| IBIS file created by T2B Version 16.0.0.01291   000
| Cadence Design Systems, Inc. 2011
| This Model is valid for  Temperature Range -40C<=Tc<=125C
| Valid for LPDDR4-1600/2400/3200 operation
| Part Number   VDD2/VDDQ   Package   Architecture
| SCE11N4G320AF   1.1 +0.07/-0.04V   BGA200   16Meg x 16 x 8 x2
| SCE11N8G322AF   1.1 +0.07/-0.04V   BGA200   32Meg x 16 x 8 x2
| SCE11N4G160AF   1.1 +0.07/-0.04V   BGA200   32Meg x 16 x 8 x1
| SCE11N2G160AF   1.1 +0.07/-0.04V   BGA200   16Meg x 16 x 8 x1
| SCE11N2G320AF   1.1 +0.07/-0.04V   BGA200   8Meg x 16 x 8 x2
[IBIS ver] 5.0
[File name]  usesnxxxxaa1.ibs
[File Rev]  1.1
[Date]   2023-09-20
[Source] Simulation of a silicon level SPICE model
[Notes]  IBIS Characteristics for I/O Buffer
   IBIS Model Revision History:
   Rev 1.0:   2020-05-11 - IBIS model file initial creation
   Rev 1.1:   2023-09-20 - update odt data
[Disclaimer]  The IBIS models are for modeling purpose only and are
   subject to change without any notice. UniIC is not
   responsible for any problems the models may cause.
[Copyright] Copyright 2023 UniIC Semiconductors Corp. All rights reserved
|   Component SCE11N4G320AF
[Component] SCE11N4G320AF
[Manufacturer] UniIC Semiconductors Corp.
[Package]
| variable   typ   min   max
R_pkg   1.150   0.687   2.340
L_pkg   1.020nH   0.634nH   2.010nH
C_pkg   0.923pF   0.644pF   3.990pF
[Pin]  signal_name   model_name   R_pin   L_pin   C_pin
A3   VSS   GND   NA   NA   NA
A4   VDD2   POWER   NA   NA   NA
A5   ZQ0   POWER   NA   NA   NA
A9   VDD2   POWER   NA   NA   NA
A10   VSS   GND   NA   NA   NA
A11   ERR_A   ERR   0.862   0.865nH   0.750pF
B2   DQ0_A   DQ   0.711   0.690nH   0.657pF
B3   VDDQ   POWER   NA   NA   NA
B4   DQ7_A   DQ   0.730   0.686nH   0.659pF
B5   VDDQ   POWER   NA   NA   NA
B8   VDDQ   POWER   NA   NA   NA
B9   DQ15_A   DQ   0.702   0.664nH   0.672pF
B10   VDDDQ   POWER   NA   NA   NA
B11   DQ8_A   DQ   0.723   0.706nH   0.669pF
C1   VSS   GND   NA   NA   NA
C2   DQ1_A   DQ   0.687   0.642nH   0.680pF
C3   DMI0_A   DQ   0.822   0.743nH   0.733pF
C4   DQ6_A   DQ   0.704   0.658nH   0.667pF
C5   VSS   GND   NA   NA   NA
C8   VSS   GND   NA   NA   NA
C9   DQ14_A   DQ   0.694   0.654nH   0.669pF
C10   DMI1_A   DQ   0.687   1.080nH   0.781pF
C11   DQ9_A   DQ   1.270   0.643nH   0.670pF
C12   VSS   GND   NA   NA   NA
D1   VDDQ   POWER   NA   NA   NA
D2   VSS   GND   NA   NA   NA
D3   DQS0_T_A   DQ   0.724   0.699nH   0.652pF
D4   VSS   GND   NA   NA   NA
D5   VDDQ   POWER   NA   NA   NA
D8   VDDQ   POWER   NA   NA   NA
D9   VSS   GND   NA   NA   NA
D10   DQS1_T_A   DQ   0.720   0.700nH   0.665pF
D11   VSS   GND   NA   NA   NA
D12   VDDQ   POWER   NA   NA   NA
E1   VSS   GND   NA   NA   NA
E2   DQ2_A   DQ   0.701   0.640nH   0.661pF
E3   DQS0_C_A   DQ   0.735   0.740nH   0.655pF
E4   DQ5_A   DQ   0.732   0.690nH   0.662pF
E5   VSS   GND   NA   NA   NA
E8   VSS   GND   NA   NA   NA
E9   DQ13_A   DQ   0.727   0.687nH   0.670pF
E10   DQS1_C_A   DQ   0.741   0.747nH   0.656pF
E11   DQ10_A   DQ   0.697   0.634nH   0.691pF
E12   VSS   GND   NA   NA   NA
F1   VDD1   POWER   NA   NA   NA
F2   DQ3_A   DQ   0.741   0.703nH   0.646pF
F3   VDDQ   POWER   NA   NA   NA
F4   DQ4_A   DQ   0.729   0.671nH   0.649pF
F5   VDD2   POWER   NA   NA   NA
F8   VDD2   POWER   NA   NA   NA
F9   DQ12_A   DQ   1.100   0.858nH   0.709pF
F10   VDDQ   POWER   NA   NA   NA
F11   DQ11_A   DQ   0.728   0.685nH   0.658pF
F12   VDD1   POWER   NA   NA   NA
G1   VSS   GND   NA   NA   NA
G2   ODT_CA_A   PINEN   1.660   1.430nH   1.024pF
G3   VSS   GND   NA   NA   NA
G4   VDD1   POWER   NA   NA   NA
G5   VSS   GND   NA   NA   NA
G8   VSS   GND   NA   NA   NA
G9   VDD1   POWER   NA   NA   NA
G10   VSS   GND   NA   NA   NA
G12   VSS   GND   NA   NA   NA
H1   VDD2   POWER   NA   NA   NA
H2   CA0_A   CLKCA   2.000   1.690nH   1.170pF
H4   CS0_A   CLKCA   1.680   1.430nH   1.070pF
H5   VDD2   POWER   NA   NA   NA
H8   VDD2   POWER   NA   NA   NA
H9   CA2_A   CLKCA   1.960   1.660nH   1.160pF
H10   CA3_A   CLKCA   1.940   1.640nH   1.170pF
H11   CA4_A   CLKCA   2.020   1.700nH   1.200pF
H12   VDD2   POWER   NA   NA   NA
J1   VSS   GND   NA   NA   NA
J2   CA1_A   CLKCA   2.000   1.680nH   1.160pF
J3   VSS   GND   NA   NA   NA
J4   CKE0_A   PINEN   1.600   1.380nH   1.000pF
J8   CK_T_A   CLKCA   1.720   1.510nH   1.050pF
J9   CK_C_A   CLKCA   1.740   1.543nH   1.050pF
J10   VSS   GND   NA   NA   NA
J11   CA5_A   CLKCA   2.030   1.690nH   1.200pF
J12   VSS   GND   NA   NA   NA
K1   VDD2   POWER   NA   NA   NA
K2   VSS   GND   NA   NA   NA
K3   VDD2   POWER   NA   NA   NA
K4   VSS   GND   NA   NA   NA
K9   VSS   GND   NA   NA   NA
K10   VDD2   POWER   NA   NA   NA
K11   VSS   GND   NA   NA   NA
K12   VDD2   POWER   NA   NA   NA
N1   VDD2   POWER   NA   NA   NA
N2   VSS   GND   NA   NA   NA
N3   VDD2   POWER   NA   NA   NA
N4   VSS   GND   NA   NA   NA
N9   VSS   GND   NA   NA   NA
N10   VDD2   POWER   NA   NA   NA
N11   VSS   GND   NA   NA   NA
N12   VDD2   POWER   NA   NA   NA
P1   VSS   GND   NA   NA   NA
P2   CA1_B   CLKCA   2.000   1.690nH   1.160pF
P3   VSS   GND   NA   NA   NA
P4   CKE0_B   PINEN   1.600   1.390nH   0.999pF
P8   CK_T_B   CLKCA   1.740   1.510nH   1.060pF
P9   CK_C_B   CLKCA   1.740   1.530nH   1.050pF
P10   VSS   GND   NA   NA   NA
P11   CA5_B   CLKCA   2.030   1.710nH   1.180pF
P12   VSS   GND   NA   NA   NA
R1   VDD2   POWER   NA   NA   NA
R2   CA0_B   CLKCA   2.000   1.690nH   1.170pF
R4   CS0_B   CLKCA   1.680   1.430nH   1.070pF
R5   VDD2   POWER   NA   NA   NA
R8   VDD2   POWER   NA   NA   NA
R9   CA2_B   CLKCA   2.000   1.700nH   1.180pF
R10   CA3_B   CLKCA   1.930   1.630nH   1.170pF
R11   CA4_B   CLKCA   1.980   1.680nH   1.190pF
R12   VDD2   POWER   NA   NA   NA
T1   VSS   GND   NA   NA   NA
T2   ODT_CA_B   PINEN   2.020   1.598nH   1.079pF
T3   VSS   GND   NA   NA   NA
T4   VDD1   POWER   NA   NA   NA
T5   VSS   GND   NA   NA   NA
T8   VSS   GND   NA   NA   NA
T9   VDD1   POWER   NA   NA   NA
T10   VSS   GND   NA   NA   NA
T11   RESET_N   PINEN   2.020   1.598nH   1.079pF
T12   VSS   GND   NA   NA   NA
U1   VDD1   POWER   NA   NA   NA
U2   DQ3_B   DQ   1.110   0.889nH   0.704pF
U3   VDDQ   POWER   NA   NA   NA
U4   DQ4_B   DQ   1.080   0.845nH   0.704pF
U5   VDD2   POWER   NA   NA   NA
U8   VDD2   POWER   NA   NA   NA
U9   DQ12_B   DQ   0.727   0.672nH   0.654pF
U10   VDDQ   POWER   NA   NA   NA
U11   DQ11_B   DQ   0.749   0.707nH   0.644pF
U12   VDD1   POWER   NA   NA   NA
V1   VSS   GND   NA   NA   NA
V2   DQ2_B   DQ   0.704   0.646nH   0.659pF
V3   DQS0_C_B   DQ   0.738   0.745nH   0.673pF
V4   DQ5_B   DQ   0.723   0.684nH   0.677pF
V5   VSS   GND   NA   NA   NA
V8   VSS   GND   NA   NA   NA
V9   DQ13_B   DQ   0.722   0.685nH   0.673pF
V10   DQS1_C_B   DQ   0.738   0.747nH   0.647pF
V11   DQ10_B   DQ   0.696   0.645nH   0.666pF
V12   VSS   GND   NA   NA   NA
W1   VDDQ   POWER   NA   NA   NA
W2   VSS   GND   NA   NA   NA
W3   DQS0_T_B   DQ   0.734   0.716nH   0.652pF
W4   VSS   GND   NA   NA   NA
W5   VDDQ   POWER   NA   NA   NA
W8   VDDQ   POWER   NA   NA   NA
W9   VSS   GND   NA   NA   NA
W10   DQS1_T_B   DQ   0.731   0.708nH   0.656pF
W11   VSS   GND   NA   NA   NA
W12   VDDQ   POWER   NA   NA   NA
Y1   VSS   GND   NA   NA   NA
Y2   DQ1_B   DQ   1.130   0.969nH   0.723pF
Y3   DMI0_B   DQ   0.820   0.739nH   0.734pF
Y4   DQ6_B   DQ   0.698   0.655nH   0.668pF
Y5   VSS   GND   NA   NA   NA
Y8   VSS   GND   NA   NA   NA
Y9   DQ14_B   DQ   0.691   0.653nH   0.672pF
Y10   DMI1_B   DQ   0.819   0.738nH   0.735pF
Y11   DQ9_B   DQ   0.688   0.642nH   0.676pF
Y12   VSS   GND   NA   NA   NA
AA2   DQ0_B   DQ   0.709   0.697nH   0.668pF
AA3   VDDQ   POWER   NA   NA   NA
AA4   DQ7_B   DQ   0.735   0.700nH   0.660pF
AA5   VDDQ   POWER   NA   NA   NA
AA8   VDDQ   POWER   NA   NA   NA
AA9   DQ15_B   DQ   0.709   0.666nH   0.683pF
AA10   VDDQ   POWER   NA   NA   NA
AA11   DQ8_B   DQ   0.716   0.695nH   0.675pF
AB3   VSS   GND   NA   NA   NA
AB4   VDD2   POWER   NA   NA   NA
AB5   VSS   GND   NA   NA   NA
AB8   VSS   GND   NA   NA   NA
AB9   VDD2   POWER   NA   NA   NA
AB10   VSS   GND   NA   NA   NA
AB11   ERR_B   ERR   2.340   2.010nH   3.990pF
|IN   dq_in   dummy
|EN   dq_en   dummy
[Diff pin]  inv_pin  vdiff   tdelay_typ   tdelay_min   tdelay_max
D3   E3   0.180V   NA   NA   NA
D10   E10   0.180V   NA   NA   NA
J8   J9   0.180V   NA   NA   NA
P8   P9   0.180V   NA   NA   NA
W3   V3   0.180V   NA   NA   NA
W10   V10   0.180V   NA   NA   NA
|   Component SCE11N8G322AF
[Component] SCE11N8G322AF
[Manufacturer] UniIC Semiconductors Corp.
[Package]
| variable   typ   min   max
R_pkg   1.150   0.687   2.340
L_pkg   1.020nH   0.634nH   2.010nH
C_pkg   0.923pF   0.644pF   3.990pF
[Pin]  signal_name   model_name   R_pin   L_pin   C_pin
A3   VSS   GND   NA   NA   NA
A4   VDD2   POWER   NA   NA   NA
A5   ZQ0   POWER   NA   NA   NA
A9   VDD2   POWER   NA   NA   NA
A10   VSS   GND   NA   NA   NA
A11   ERR_A   ERR   0.862   0.865nH   0.750pF
B2   DQ0_A   DQ   0.711   0.690nH   0.657pF
B3   VDDQ   POWER   NA   NA   NA
B4   DQ7_A   DQ   0.730   0.686nH   0.659pF
B5   VDDQ   POWER   NA   NA   NA
B8   VDDQ   POWER   NA   NA   NA
B9   DQ15_A   DQ   0.702   0.664nH   0.672pF
B10   VDDDQ   POWER   NA   NA   NA
B11   DQ8_A   DQ   0.723   0.706nH   0.669pF
C1   VSS   GND   NA   NA   NA
C2   DQ1_A   DQ   0.687   0.642nH   0.680pF
C3   DMI0_A   DQ   0.822   0.743nH   0.733pF
C4   DQ6_A   DQ   0.704   0.658nH   0.667pF
C5   VSS   GND   NA   NA   NA
C8   VSS   GND   NA   NA   NA
C9   DQ14_A   DQ   0.694   0.654nH   0.669pF
C10   DMI1_A   DQ   0.687   1.080nH   0.781pF
C11   DQ9_A   DQ   1.270   0.643nH   0.670pF
C12   VSS   GND   NA   NA   NA
D1   VDDQ   POWER   NA   NA   NA
D2   VSS   GND   NA   NA   NA
D3   DQS0_T_A   DQ   0.724   0.699nH   0.652pF
D4   VSS   GND   NA   NA   NA
D5   VDDQ   POWER   NA   NA   NA
D8   VDDQ   POWER   NA   NA   NA
D9   VSS   GND   NA   NA   NA
D10   DQS1_T_A   DQ   0.720   0.700nH   0.665pF
D11   VSS   GND   NA   NA   NA
D12   VDDQ   POWER   NA   NA   NA
E1   VSS   GND   NA   NA   NA
E2   DQ2_A   DQ   0.701   0.640nH   0.661pF
E3   DQS0_C_A   DQ   0.735   0.740nH   0.655pF
E4   DQ5_A   DQ   0.732   0.690nH   0.662pF
E5   VSS   GND   NA   NA   NA
E8   VSS   GND   NA   NA   NA
E9   DQ13_A   DQ   0.727   0.687nH   0.670pF
E10   DQS1_C_A   DQ   0.741   0.747nH   0.656pF
E11   DQ10_A   DQ   0.697   0.634nH   0.691pF
E12   VSS   GND   NA   NA   NA
F1   VDD1   POWER   NA   NA   NA
F2   DQ3_A   DQ   0.741   0.703nH   0.646pF
F3   VDDQ   POWER   NA   NA   NA
F4   DQ4_A   DQ   0.729   0.671nH   0.649pF
F5   VDD2   POWER   NA   NA   NA
F8   VDD2   POWER   NA   NA   NA
F9   DQ12_A   DQ   1.100   0.858nH   0.709pF
F10   VDDQ   POWER   NA   NA   NA
F11   DQ11_A   DQ   0.728   0.685nH   0.658pF
F12   VDD1   POWER   NA   NA   NA
G1   VSS   GND   NA   NA   NA
G2   ODT_CA_A   PINEN   1.660   1.430nH   1.024pF
G3   VSS   GND   NA   NA   NA
G4   VDD1   POWER   NA   NA   NA
G5   VSS   GND   NA   NA   NA
G8   VSS   GND   NA   NA   NA
G9   VDD1   POWER   NA   NA   NA
G10   VSS   GND   NA   NA   NA
G12   VSS   GND   NA   NA   NA
H1   VDD2   POWER   NA   NA   NA
H2   CA0_A   CLKCA   2.000   1.690nH   1.170pF
H4   CS0_A   CLKCA   1.680   1.430nH   1.070pF
H5   VDD2   POWER   NA   NA   NA
H8   VDD2   POWER   NA   NA   NA
H9   CA2_A   CLKCA   1.960   1.660nH   1.160pF
H10   CA3_A   CLKCA   1.940   1.640nH   1.170pF
H11   CA4_A   CLKCA   2.020   1.700nH   1.200pF
H12   VDD2   POWER   NA   NA   NA
J1   VSS   GND   NA   NA   NA
J2   CA1_A   CLKCA   2.000   1.680nH   1.160pF
J3   VSS   GND   NA   NA   NA
J4   CKE0_A   PINEN   1.600   1.380nH   1.000pF
J8   CK_T_A   CLKCA   1.720   1.510nH   1.050pF
J9   CK_C_A   CLKCA   1.740   1.543nH   1.050pF
J10   VSS   GND   NA   NA   NA
J11   CA5_A   CLKCA   2.030   1.690nH   1.200pF
J12   VSS   GND   NA   NA   NA
K1   VDD2   POWER   NA   NA   NA
K2   VSS   GND   NA   NA   NA
K3   VDD2   POWER   NA   NA   NA
K4   VSS   GND   NA   NA   NA
K9   VSS   GND   NA   NA   NA
K10   VDD2   POWER   NA   NA   NA
K11   VSS   GND   NA   NA   NA
K12   VDD2   POWER   NA   NA   NA
N1   VDD2   POWER   NA   NA   NA
N2   VSS   GND   NA   NA   NA
N3   VDD2   POWER   NA   NA   NA
N4   VSS   GND   NA   NA   NA
N9   VSS   GND   NA   NA   NA
N10   VDD2   POWER   NA   NA   NA
N11   VSS   GND   NA   NA   NA
N12   VDD2   POWER   NA   NA   NA
P1   VSS   GND   NA   NA   NA
P2   CA1_B   CLKCA   2.000   1.690nH   1.160pF
P3   VSS   GND   NA   NA   NA
P4   CKE0_B   PINEN   1.600   1.390nH   0.999pF
P8   CK_T_B   CLKCA   1.740   1.510nH   1.060pF
P9   CK_C_B   CLKCA   1.740   1.530nH   1.050pF
P10   VSS   GND   NA   NA   NA
P11   CA5_B   CLKCA   2.030   1.710nH   1.180pF
P12   VSS   GND   NA   NA   NA
R1   VDD2   POWER   NA   NA   NA
R2   CA0_B   CLKCA   2.000   1.690nH   1.170pF
R4   CS0_B   CLKCA   1.680   1.430nH   1.070pF
R5   VDD2   POWER   NA   NA   NA
R8   VDD2   POWER   NA   NA   NA
R9   CA2_B   CLKCA   2.000   1.700nH   1.180pF
R10   CA3_B   CLKCA   1.930   1.630nH   1.170pF
R11   CA4_B   CLKCA   1.980   1.680nH   1.190pF
R12   VDD2   POWER   NA   NA   NA
T1   VSS   GND   NA   NA   NA
T2   ODT_CA_B   PINEN   2.020   1.598nH   1.079pF
T3   VSS   GND   NA   NA   NA
T4   VDD1   POWER   NA   NA   NA
T5   VSS   GND   NA   NA   NA
T8   VSS   GND   NA   NA   NA
T9   VDD1   POWER   NA   NA   NA
T10   VSS   GND   NA   NA   NA
T11   RESET_N   PINEN   2.020   1.598nH   1.079pF
T12   VSS   GND   NA   NA   NA
U1   VDD1   POWER   NA   NA   NA
U2   DQ3_B   DQ   1.110   0.889nH   0.704pF
U3   VDDQ   POWER   NA   NA   NA
U4   DQ4_B   DQ   1.080   0.845nH   0.704pF
U5   VDD2   POWER   NA   NA   NA
U8   VDD2   POWER   NA   NA   NA
U9   DQ12_B   DQ   0.727   0.672nH   0.654pF
U10   VDDQ   POWER   NA   NA   NA
U11   DQ11_B   DQ   0.749   0.707nH   0.644pF
U12   VDD1   POWER   NA   NA   NA
V1   VSS   GND   NA   NA   NA
V2   DQ2_B   DQ   0.704   0.646nH   0.659pF
V3   DQS0_C_B   DQ   0.738   0.745nH   0.673pF
V4   DQ5_B   DQ   0.723   0.684nH   0.677pF
V5   VSS   GND   NA   NA   NA
V8   VSS   GND   NA   NA   NA
V9   DQ13_B   DQ   0.722   0.685nH   0.673pF
V10   DQS1_C_B   DQ   0.738   0.747nH   0.647pF
V11   DQ10_B   DQ   0.696   0.645nH   0.666pF
V12   VSS   GND   NA   NA   NA
W1   VDDQ   POWER   NA   NA   NA
W2   VSS   GND   NA   NA   NA
W3   DQS0_T_B   DQ   0.734   0.716nH   0.652pF
W4   VSS   GND   NA   NA   NA
W5   VDDQ   POWER   NA   NA   NA
W8   VDDQ   POWER   NA   NA   NA
W9   VSS   GND   NA   NA   NA
W10   DQS1_T_B   DQ   0.731   0.708nH   0.656pF
W11   VSS   GND   NA   NA   NA
W12   VDDQ   POWER   NA   NA   NA
Y1   VSS   GND   NA   NA   NA
Y2   DQ1_B   DQ   1.130   0.969nH   0.723pF
Y3   DMI0_B   DQ   0.820   0.739nH   0.734pF
Y4   DQ6_B   DQ   0.698   0.655nH   0.668pF
Y5   VSS   GND   NA   NA   NA
Y8   VSS   GND   NA   NA   NA
Y9   DQ14_B   DQ   0.691   0.653nH   0.672pF
Y10   DMI1_B   DQ   0.819   0.738nH   0.735pF
Y11   DQ9_B   DQ   0.688   0.642nH   0.676pF
Y12   VSS   GND   NA   NA   NA
AA2   DQ0_B   DQ   0.709   0.697nH   0.668pF
AA3   VDDQ   POWER   NA   NA   NA
AA4   DQ7_B   DQ   0.735   0.700nH   0.660pF
AA5   VDDQ   POWER   NA   NA   NA
AA8   VDDQ   POWER   NA   NA   NA
AA9   DQ15_B   DQ   0.709   0.666nH   0.683pF
AA10   VDDQ   POWER   NA   NA   NA
AA11   DQ8_B   DQ   0.716   0.695nH   0.675pF
AB3   VSS   GND   NA   NA   NA
AB4   VDD2   POWER   NA   NA   NA
AB5   VSS   GND   NA   NA   NA
AB8   VSS   GND   NA   NA   NA
AB9   VDD2   POWER   NA   NA   NA
AB10   VSS   GND   NA   NA   NA
AB11   ERR_B   ERR   2.340   2.010nH   3.990pF
|IN   dq_in   dummy
|EN   dq_en   dummy
[Diff pin]  inv_pin  vdiff   tdelay_typ   tdelay_min   tdelay_max
D3   E3   0.180V   NA   NA   NA
D10   E10   0.180V   NA   NA   NA
J8   J9   0.180V   NA   NA   NA
P8   P9   0.180V   NA   NA   NA
W3   V3   0.180V   NA   NA   NA
W10   V10   0.180V   NA   NA   NA
|   Component SCE11N4G160AF
[Component] SCE11N4G160AF
[Manufacturer] UniIC Semiconductors Corp.
[Package]
| variable   typ   min   max
R_pkg   1.150   0.687   2.340
L_pkg   1.020nH   0.634nH   2.010nH
C_pkg   0.923pF   0.644pF   3.990pF
[Pin]  signal_name   model_name   R_pin   L_pin   C_pin
A3   VSS   GND   NA   NA   NA
A4   VDD2   POWER   NA   NA   NA
A5   ZQ0   POWER   NA   NA   NA
A9   VDD2   POWER   NA   NA   NA
A10   VSS   GND   NA   NA   NA
A11   ERR_A   ERR   0.862   0.865nH   0.750pF
B2   DQ0_A   DQ   0.711   0.690nH   0.657pF
B3   VDDQ   POWER   NA   NA   NA
B4   DQ7_A   DQ   0.730   0.686nH   0.659pF
B5   VDDQ   POWER   NA   NA   NA
B8   VDDQ   POWER   NA   NA   NA
B9   DQ15_A   DQ   0.702   0.664nH   0.672pF
B10   VDDDQ   POWER   NA   NA   NA
B11   DQ8_A   DQ   0.723   0.706nH   0.669pF
C1   VSS   GND   NA   NA   NA
C2   DQ1_A   DQ   0.687   0.642nH   0.680pF
C3   DMI0_A   DQ   0.822   0.743nH   0.733pF
C4   DQ6_A   DQ   0.704   0.658nH   0.667pF
C5   VSS   GND   NA   NA   NA
C8   VSS   GND   NA   NA   NA
C9   DQ14_A   DQ   0.694   0.654nH   0.669pF
C10   DMI1_A   DQ   0.687   1.080nH   0.781pF
C11   DQ9_A   DQ   1.270   0.643nH   0.670pF
C12   VSS   GND   NA   NA   NA
D1   VDDQ   POWER   NA   NA   NA
D2   VSS   GND   NA   NA   NA
D3   DQS0_T_A   DQ   0.724   0.699nH   0.652pF
D4   VSS   GND   NA   NA   NA
D5   VDDQ   POWER   NA   NA   NA
D8   VDDQ   POWER   NA   NA   NA
D9   VSS   GND   NA   NA   NA
D10   DQS1_T_A   DQ   0.720   0.700nH   0.665pF
D11   VSS   GND   NA   NA   NA
D12   VDDQ   POWER   NA   NA   NA
E1   VSS   GND   NA   NA   NA
E2   DQ2_A   DQ   0.701   0.640nH   0.661pF
E3   DQS0_C_A   DQ   0.735   0.740nH   0.655pF
E4   DQ5_A   DQ   0.732   0.690nH   0.662pF
E5   VSS   GND   NA   NA   NA
E8   VSS   GND   NA   NA   NA
E9   DQ13_A   DQ   0.727   0.687nH   0.670pF
E10   DQS1_C_A   DQ   0.741   0.747nH   0.656pF
E11   DQ10_A   DQ   0.697   0.634nH   0.691pF
E12   VSS   GND   NA   NA   NA
F1   VDD1   POWER   NA   NA   NA
F2   DQ3_A   DQ   0.741   0.703nH   0.646pF
F3   VDDQ   POWER   NA   NA   NA
F4   DQ4_A   DQ   0.729   0.671nH   0.649pF
F5   VDD2   POWER   NA   NA   NA
F8   VDD2   POWER   NA   NA   NA
F9   DQ12_A   DQ   1.100   0.858nH   0.709pF
F10   VDDQ   POWER   NA   NA   NA
F11   DQ11_A   DQ   0.728   0.685nH   0.658pF
F12   VDD1   POWER   NA   NA   NA
G1   VSS   GND   NA   NA   NA
G2   ODT_CA_A   PINEN   1.660   1.430nH   1.024pF
G3   VSS   GND   NA   NA   NA
G4   VDD1   POWER   NA   NA   NA
G5   VSS   GND   NA   NA   NA
G8   VSS   GND   NA   NA   NA
G9   VDD1   POWER   NA   NA   NA
G10   VSS   GND   NA   NA   NA
G12   VSS   GND   NA   NA   NA
H1   VDD2   POWER   NA   NA   NA
H2   CA0_A   CLKCA   2.000   1.690nH   1.170pF
H4   CS0_A   CLKCA   1.680   1.430nH   1.070pF
H5   VDD2   POWER   NA   NA   NA
H8   VDD2   POWER   NA   NA   NA
H9   CA2_A   CLKCA   1.960   1.660nH   1.160pF
H10   CA3_A   CLKCA   1.940   1.640nH   1.170pF
H11   CA4_A   CLKCA   2.020   1.700nH   1.200pF
H12   VDD2   POWER   NA   NA   NA
J1   VSS   GND   NA   NA   NA
J2   CA1_A   CLKCA   2.000   1.680nH   1.160pF
J3   VSS   GND   NA   NA   NA
J4   CKE0_A   PINEN   1.600   1.380nH   1.000pF
J8   CK_T_A   CLKCA   1.720   1.510nH   1.050pF
J9   CK_C_A   CLKCA   1.740   1.543nH   1.050pF
J10   VSS   GND   NA   NA   NA
J11   CA5_A   CLKCA   2.030   1.690nH   1.200pF
J12   VSS   GND   NA   NA   NA
K1   VDD2   POWER   NA   NA   NA
K2   VSS   GND   NA   NA   NA
K3   VDD2   POWER   NA   NA   NA
K4   VSS   GND   NA   NA   NA
K9   VSS   GND   NA   NA   NA
K10   VDD2   POWER   NA   NA   NA
K11   VSS   GND   NA   NA   NA
K12   VDD2   POWER   NA   NA   NA
N1   VDD2   POWER   NA   NA   NA
N2   VSS   GND   NA   NA   NA
N3   VDD2   POWER   NA   NA   NA
N4   VSS   GND   NA   NA   NA
N9   VSS   GND   NA   NA   NA
N10   VDD2   POWER   NA   NA   NA
N11   VSS   GND   NA   NA   NA
N12   VDD2   POWER   NA   NA   NA
P1   VSS   GND   NA   NA   NA
P3   VSS   GND   NA   NA   NA
P10   VSS   GND   NA   NA   NA
P12   VSS   GND   NA   NA   NA
R1   VDD2   POWER   NA   NA   NA
R5   VDD2   POWER   NA   NA   NA
R8   VDD2   POWER   NA   NA   NA
R12   VDD2   POWER   NA   NA   NA
T1   VSS   GND   NA   NA   NA
T3   VSS   GND   NA   NA   NA
T4   VDD1   POWER   NA   NA   NA
T5   VSS   GND   NA   NA   NA
T8   VSS   GND   NA   NA   NA
T9   VDD1   POWER   NA   NA   NA
T10   VSS   GND   NA   NA   NA
T11   RESET_N   PINEN   2.020   1.598nH   1.079pF
T12   VSS   GND   NA   NA   NA
U1   VDD1   POWER   NA   NA   NA
U3   VDDQ   POWER   NA   NA   NA
U5   VDD2   POWER   NA   NA   NA
U8   VDD2   POWER   NA   NA   NA
U10   VDDQ   POWER   NA   NA   NA
U12   VDD1   POWER   NA   NA   NA
V1   VSS   GND   NA   NA   NA
V5   VSS   GND   NA   NA   NA
V8   VSS   GND   NA   NA   NA
V12   VSS   GND   NA   NA   NA
W1   VDDQ   POWER   NA   NA   NA
W2   VSS   GND   NA   NA   NA
W4   VSS   GND   NA   NA   NA
W5   VDDQ   POWER   NA   NA   NA
W8   VDDQ   POWER   NA   NA   NA
W9   VSS   GND   NA   NA   NA
W11   VSS   GND   NA   NA   NA
W12   VDDQ   POWER   NA   NA   NA
Y1   VSS   GND   NA   NA   NA
Y5   VSS   GND   NA   NA   NA
Y8   VSS   GND   NA   NA   NA
Y12   VSS   GND   NA   NA   NA
AA3   VDDQ   POWER   NA   NA   NA
AA5   VDDQ   POWER   NA   NA   NA
AA8   VDDQ   POWER   NA   NA   NA
AA10   VDDQ   POWER   NA   NA   NA
AB3   VSS   GND   NA   NA   NA
AB4   VDD2   POWER   NA   NA   NA
AB5   VSS   GND   NA   NA   NA
AB8   VSS   GND   NA   NA   NA
AB9   VDD2   POWER   NA   NA   NA
AB10   VSS   GND   NA   NA   NA
|IN   dq_in   dummy
|EN   dq_en   dummy
[Diff pin]  inv_pin  vdiff   tdelay_typ   tdelay_min   tdelay_max
D3   E3   0.180V   NA   NA   NA
D10   E10   0.180V   NA   NA   NA
J8   J9   0.180V   NA   NA   NA
|   Component SCE11N2G160AF
[Component] SCE11N2G160AF
[Manufacturer] UniIC Semiconductors Corp.
[Package]
| variable   typ   min   max
R_pkg   1.150   0.687   2.340
L_pkg   1.020nH   0.634nH   2.010nH
C_pkg   0.923pF   0.644pF   3.990pF
[Pin]  signal_name   model_name   R_pin   L_pin   C_pin
A3   VSS   GND   NA   NA   NA
A4   VDD2   POWER   NA   NA   NA
A5   ZQ0   POWER   NA   NA   NA
A9   VDD2   POWER   NA   NA   NA
A10   VSS   GND   NA   NA   NA
A11   ERR_A   ERR   0.862   0.865nH   0.750pF
B2   DQ0_A   DQ   0.711   0.690nH   0.657pF
B3   VDDQ   POWER   NA   NA   NA
B4   DQ7_A   DQ   0.730   0.686nH   0.659pF
B5   VDDQ   POWER   NA   NA   NA
B8   VDDQ   POWER   NA   NA   NA
B9   DQ15_A   DQ   0.702   0.664nH   0.672pF
B10   VDDDQ   POWER   NA   NA   NA
B11   DQ8_A   DQ   0.723   0.706nH   0.669pF
C1   VSS   GND   NA   NA   NA
C2   DQ1_A   DQ   0.687   0.642nH   0.680pF
C3   DMI0_A   DQ   0.822   0.743nH   0.733pF
C4   DQ6_A   DQ   0.704   0.658nH   0.667pF
C5   VSS   GND   NA   NA   NA
C8   VSS   GND   NA   NA   NA
C9   DQ14_A   DQ   0.694   0.654nH   0.669pF
C10   DMI1_A   DQ   0.687   1.080nH   0.781pF
C11   DQ9_A   DQ   1.270   0.643nH   0.670pF
C12   VSS   GND   NA   NA   NA
D1   VDDQ   POWER   NA   NA   NA
D2   VSS   GND   NA   NA   NA
D3   DQS0_T_A   DQ   0.724   0.699nH   0.652pF
D4   VSS   GND   NA   NA   NA
D5   VDDQ   POWER   NA   NA   NA
D8   VDDQ   POWER   NA   NA   NA
D9   VSS   GND   NA   NA   NA
D10   DQS1_T_A   DQ   0.720   0.700nH   0.665pF
D11   VSS   GND   NA   NA   NA
D12   VDDQ   POWER   NA   NA   NA
E1   VSS   GND   NA   NA   NA
E2   DQ2_A   DQ   0.701   0.640nH   0.661pF
E3   DQS0_C_A   DQ   0.735   0.740nH   0.655pF
E4   DQ5_A   DQ   0.732   0.690nH   0.662pF
E5   VSS   GND   NA   NA   NA
E8   VSS   GND   NA   NA   NA
E9   DQ13_A   DQ   0.727   0.687nH   0.670pF
E10   DQS1_C_A   DQ   0.741   0.747nH   0.656pF
E11   DQ10_A   DQ   0.697   0.634nH   0.691pF
E12   VSS   GND   NA   NA   NA
F1   VDD1   POWER   NA   NA   NA
F2   DQ3_A   DQ   0.741   0.703nH   0.646pF
F3   VDDQ   POWER   NA   NA   NA
F4   DQ4_A   DQ   0.729   0.671nH   0.649pF
F5   VDD2   POWER   NA   NA   NA
F8   VDD2   POWER   NA   NA   NA
F9   DQ12_A   DQ   1.100   0.858nH   0.709pF
F10   VDDQ   POWER   NA   NA   NA
F11   DQ11_A   DQ   0.728   0.685nH   0.658pF
F12   VDD1   POWER   NA   NA   NA
G1   VSS   GND   NA   NA   NA
G2   ODT_CA_A   PINEN   1.660   1.430nH   1.024pF
G3   VSS   GND   NA   NA   NA
G4   VDD1   POWER   NA   NA   NA
G5   VSS   GND   NA   NA   NA
G8   VSS   GND   NA   NA   NA
G9   VDD1   POWER   NA   NA   NA
G10   VSS   GND   NA   NA   NA
G12   VSS   GND   NA   NA   NA
H1   VDD2   POWER   NA   NA   NA
H2   CA0_A   CLKCA   2.000   1.690nH   1.170pF
H4   CS0_A   CLKCA   1.680   1.430nH   1.070pF
H5   VDD2   POWER   NA   NA   NA
H8   VDD2   POWER   NA   NA   NA
H9   CA2_A   CLKCA   1.960   1.660nH   1.160pF
H10   CA3_A   CLKCA   1.940   1.640nH   1.170pF
H11   CA4_A   CLKCA   2.020   1.700nH   1.200pF
H12   VDD2   POWER   NA   NA   NA
J1   VSS   GND   NA   NA   NA
J2   CA1_A   CLKCA   2.000   1.680nH   1.160pF
J3   VSS   GND   NA   NA   NA
J4   CKE0_A   PINEN   1.600   1.380nH   1.000pF
J8   CK_T_A   CLKCA   1.720   1.510nH   1.050pF
J9   CK_C_A   CLKCA   1.740   1.543nH   1.050pF
J10   VSS   GND   NA   NA   NA
J11   CA5_A   CLKCA   2.030   1.690nH   1.200pF
J12   VSS   GND   NA   NA   NA
K1   VDD2   POWER   NA   NA   NA
K2   VSS   GND   NA   NA   NA
K3   VDD2   POWER   NA   NA   NA
K4   VSS   GND   NA   NA   NA
K9   VSS   GND   NA   NA   NA
K10   VDD2   POWER   NA   NA   NA
K11   VSS   GND   NA   NA   NA
K12   VDD2   POWER   NA   NA   NA
N1   VDD2   POWER   NA   NA   NA
N2   VSS   GND   NA   NA   NA
N3   VDD2   POWER   NA   NA   NA
N4   VSS   GND   NA   NA   NA
N9   VSS   GND   NA   NA   NA
N10   VDD2   POWER   NA   NA   NA
N11   VSS   GND   NA   NA   NA
N12   VDD2   POWER   NA   NA   NA
P1   VSS   GND   NA   NA   NA
P3   VSS   GND   NA   NA   NA
P10   VSS   GND   NA   NA   NA
P12   VSS   GND   NA   NA   NA
R1   VDD2   POWER   NA   NA   NA
R5   VDD2   POWER   NA   NA   NA
R8   VDD2   POWER   NA   NA   NA
R12   VDD2   POWER   NA   NA   NA
T1   VSS   GND   NA   NA   NA
T3   VSS   GND   NA   NA   NA
T4   VDD1   POWER   NA   NA   NA
T5   VSS   GND   NA   NA   NA
T8   VSS   GND   NA   NA   NA
T9   VDD1   POWER   NA   NA   NA
T10   VSS   GND   NA   NA   NA
T11   RESET_N   PINEN   2.020   1.598nH   1.079pF
T12   VSS   GND   NA   NA   NA
U1   VDD1   POWER   NA   NA   NA
U3   VDDQ   POWER   NA   NA   NA
U5   VDD2   POWER   NA   NA   NA
U8   VDD2   POWER   NA   NA   NA
U10   VDDQ   POWER   NA   NA   NA
U12   VDD1   POWER   NA   NA   NA
V1   VSS   GND   NA   NA   NA
V5   VSS   GND   NA   NA   NA
V8   VSS   GND   NA   NA   NA
V12   VSS   GND   NA   NA   NA
W1   VDDQ   POWER   NA   NA   NA
W2   VSS   GND   NA   NA   NA
W4   VSS   GND   NA   NA   NA
W5   VDDQ   POWER   NA   NA   NA
W8   VDDQ   POWER   NA   NA   NA
W9   VSS   GND   NA   NA   NA
W11   VSS   GND   NA   NA   NA
W12   VDDQ   POWER   NA   NA   NA
Y1   VSS   GND   NA   NA   NA
Y5   VSS   GND   NA   NA   NA
Y8   VSS   GND   NA   NA   NA
Y12   VSS   GND   NA   NA   NA
AA3   VDDQ   POWER   NA   NA   NA
AA5   VDDQ   POWER   NA   NA   NA
AA8   VDDQ   POWER   NA   NA   NA
AA10   VDDQ   POWER   NA   NA   NA
AB3   VSS   GND   NA   NA   NA
AB4   VDD2   POWER   NA   NA   NA
AB5   VSS   GND   NA   NA   NA
AB8   VSS   GND   NA   NA   NA
AB9   VDD2   POWER   NA   NA   NA
AB10   VSS   GND   NA   NA   NA
|IN   dq_in   dummy
|EN   dq_en   dummy
[Diff pin]  inv_pin  vdiff   tdelay_typ   tdelay_min   tdelay_max
D3   E3   0.180V   NA   NA   NA
D10   E10   0.180V   NA   NA   NA
J8   J9   0.180V   NA   NA   NA
|   Component SCE11N2G320AF
[Component] SCE11N2G320AF
[Manufacturer] UniIC Semiconductors Corp.
[Package]
| variable   typ   min   max
R_pkg   1.150   0.687   2.340
L_pkg   1.020nH   0.634nH   2.010nH
C_pkg   0.923pF   0.644pF   3.990pF
[Pin]  signal_name   model_name   R_pin   L_pin   C_pin
A3   VSS   GND   NA   NA   NA
A4   VDD2   POWER   NA   NA   NA
A5   ZQ0   POWER   NA   NA   NA
A9   VDD2   POWER   NA   NA   NA
A10   VSS   GND   NA   NA   NA
A11   ERR_A   ERR   0.862   0.865nH   0.750pF
B2   DQ0_A   DQ   0.711   0.690nH   0.657pF
B3   VDDQ   POWER   NA   NA   NA
B4   DQ7_A   DQ   0.730   0.686nH   0.659pF
B5   VDDQ   POWER   NA   NA   NA
B8   VDDQ   POWER   NA   NA   NA
B9   DQ15_A   DQ   0.702   0.664nH   0.672pF
B10   VDDDQ   POWER   NA   NA   NA
B11   DQ8_A   DQ   0.723   0.706nH   0.669pF
C1   VSS   GND   NA   NA   NA
C2   DQ1_A   DQ   0.687   0.642nH   0.680pF
C3   DMI0_A   DQ   0.822   0.743nH   0.733pF
C4   DQ6_A   DQ   0.704   0.658nH   0.667pF
C5   VSS   GND   NA   NA   NA
C8   VSS   GND   NA   NA   NA
C9   DQ14_A   DQ   0.694   0.654nH   0.669pF
C10   DMI1_A   DQ   0.687   1.080nH   0.781pF
C11   DQ9_A   DQ   1.270   0.643nH   0.670pF
C12   VSS   GND   NA   NA   NA
D1   VDDQ   POWER   NA   NA   NA
D2   VSS   GND   NA   NA   NA
D3   DQS0_T_A   DQ   0.724   0.699nH   0.652pF
D4   VSS   GND   NA   NA   NA
D5   VDDQ   POWER   NA   NA   NA
D8   VDDQ   POWER   NA   NA   NA
D9   VSS   GND   NA   NA   NA
D10   DQS1_T_A   DQ   0.720   0.700nH   0.665pF
D11   VSS   GND   NA   NA   NA
D12   VDDQ   POWER   NA   NA   NA
E1   VSS   GND   NA   NA   NA
E2   DQ2_A   DQ   0.701   0.640nH   0.661pF
E3   DQS0_C_A   DQ   0.735   0.740nH   0.655pF
E4   DQ5_A   DQ   0.732   0.690nH   0.662pF
E5   VSS   GND   NA   NA   NA
E8   VSS   GND   NA   NA   NA
E9   DQ13_A   DQ   0.727   0.687nH   0.670pF
E10   DQS1_C_A   DQ   0.741   0.747nH   0.656pF
E11   DQ10_A   DQ   0.697   0.634nH   0.691pF
E12   VSS   GND   NA   NA   NA
F1   VDD1   POWER   NA   NA   NA
F2   DQ3_A   DQ   0.741   0.703nH   0.646pF
F3   VDDQ   POWER   NA   NA   NA
F4   DQ4_A   DQ   0.729   0.671nH   0.649pF
F5   VDD2   POWER   NA   NA   NA
F8   VDD2   POWER   NA   NA   NA
F9   DQ12_A   DQ   1.100   0.858nH   0.709pF
F10   VDDQ   POWER   NA   NA   NA
F11   DQ11_A   DQ   0.728   0.685nH   0.658pF
F12   VDD1   POWER   NA   NA   NA
G1   VSS   GND   NA   NA   NA
G2   ODT_CA_A   PINEN   1.660   1.430nH   1.024pF
G3   VSS   GND   NA   NA   NA
G4   VDD1   POWER   NA   NA   NA
G5   VSS   GND   NA   NA   NA
G8   VSS   GND   NA   NA   NA
G9   VDD1   POWER   NA   NA   NA
G10   VSS   GND   NA   NA   NA
G12   VSS   GND   NA   NA   NA
H1   VDD2   POWER   NA   NA   NA
H2   CA0_A   CLKCA   2.000   1.690nH   1.170pF
H4   CS0_A   CLKCA   1.680   1.430nH   1.070pF
H5   VDD2   POWER   NA   NA   NA
H8   VDD2   POWER   NA   NA   NA
H9   CA2_A   CLKCA   1.960   1.660nH   1.160pF
H10   CA3_A   CLKCA   1.940   1.640nH   1.170pF
H11   CA4_A   CLKCA   2.020   1.700nH   1.200pF
H12   VDD2   POWER   NA   NA   NA
J1   VSS   GND   NA   NA   NA
J2   CA1_A   CLKCA   2.000   1.680nH   1.160pF
J3   VSS   GND   NA   NA   NA
J4   CKE0_A   PINEN   1.600   1.380nH   1.000pF
J8   CK_T_A   CLKCA   1.720   1.510nH   1.050pF
J9   CK_C_A   CLKCA   1.740   1.543nH   1.050pF
J10   VSS   GND   NA   NA   NA
J11   CA5_A   CLKCA   2.030   1.690nH   1.200pF
J12   VSS   GND   NA   NA   NA
K1   VDD2   POWER   NA   NA   NA
K2   VSS   GND   NA   NA   NA
K3   VDD2   POWER   NA   NA   NA
K4   VSS   GND   NA   NA   NA
K9   VSS   GND   NA   NA   NA
K10   VDD2   POWER   NA   NA   NA
K11   VSS   GND   NA   NA   NA
K12   VDD2   POWER   NA   NA   NA
N1   VDD2   POWER   NA   NA   NA
N2   VSS   GND   NA   NA   NA
N3   VDD2   POWER   NA   NA   NA
N4   VSS   GND   NA   NA   NA
N9   VSS   GND   NA   NA   NA
N10   VDD2   POWER   NA   NA   NA
N11   VSS   GND   NA   NA   NA
N12   VDD2   POWER   NA   NA   NA
P1   VSS   GND   NA   NA   NA
P2   CA1_B   CLKCA   2.000   1.690nH   1.160pF
P3   VSS   GND   NA   NA   NA
P4   CKE0_B   PINEN   1.600   1.390nH   0.999pF
P8   CK_T_B   CLKCA   1.740   1.510nH   1.060pF
P9   CK_C_B   CLKCA   1.740   1.530nH   1.050pF
P10   VSS   GND   NA   NA   NA
P11   CA5_B   CLKCA   2.030   1.710nH   1.180pF
P12   VSS   GND   NA   NA   NA
R1   VDD2   POWER   NA   NA   NA
R2   CA0_B   CLKCA   2.000   1.690nH   1.170pF
R4   CS0_B   CLKCA   1.680   1.430nH   1.070pF
R5   VDD2   POWER   NA   NA   NA
R8   VDD2   POWER   NA   NA   NA
R9   CA2_B   CLKCA   2.000   1.700nH   1.180pF
R10   CA3_B   CLKCA   1.930   1.630nH   1.170pF
R11   CA4_B   CLKCA   1.980   1.680nH   1.190pF
R12   VDD2   POWER   NA   NA   NA
T1   VSS   GND   NA   NA   NA
T2   ODT_CA_B   PINEN   2.020   1.598nH   1.079pF
T3   VSS   GND   NA   NA   NA
T4   VDD1   POWER   NA   NA   NA
T5   VSS   GND   NA   NA   NA
T8   VSS   GND   NA   NA   NA
T9   VDD1   POWER   NA   NA   NA
T10   VSS   GND   NA   NA   NA
T11   RESET_N   PINEN   2.020   1.598nH   1.079pF
T12   VSS   GND   NA   NA   NA
U1   VDD1   POWER   NA   NA   NA
U2   DQ3_B   DQ   1.110   0.889nH   0.704pF
U3   VDDQ   POWER   NA   NA   NA
U4   DQ4_B   DQ   1.080   0.845nH   0.704pF
U5   VDD2   POWER   NA   NA   NA
U8   VDD2   POWER   NA   NA   NA
U9   DQ12_B   DQ   0.727   0.672nH   0.654pF
U10   VDDQ   POWER   NA   NA   NA
U11   DQ11_B   DQ   0.749   0.707nH   0.644pF
U12   VDD1   POWER   NA   NA   NA
V1   VSS   GND   NA   NA   NA
V2   DQ2_B   DQ   0.704   0.646nH   0.659pF
V3   DQS0_C_B   DQ   0.738   0.745nH   0.673pF
V4   DQ5_B   DQ   0.723   0.684nH   0.677pF
V5   VSS   GND   NA   NA   NA
V8   VSS   GND   NA   NA   NA
V9   DQ13_B   DQ   0.722   0.685nH   0.673pF
V10   DQS1_C_B   DQ   0.738   0.747nH   0.647pF
V11   DQ10_B   DQ   0.696   0.645nH   0.666pF
V12   VSS   GND   NA   NA   NA
W1   VDDQ   POWER   NA   NA   NA
W2   VSS   GND   NA   NA   NA
W3   DQS0_T_B   DQ   0.734   0.716nH   0.652pF
W4   VSS   GND   NA   NA   NA
W5   VDDQ   POWER   NA   NA   NA
W8   VDDQ   POWER   NA   NA   NA
W9   VSS   GND   NA   NA   NA
W10   DQS1_T_B   DQ   0.731   0.708nH   0.656pF
W11   VSS   GND   NA   NA   NA
W12   VDDQ   POWER   NA   NA   NA
Y1   VSS   GND   NA   NA   NA
Y2   DQ1_B   DQ   1.130   0.969nH   0.723pF
Y3   DMI0_B   DQ   0.820   0.739nH   0.734pF
Y4   DQ6_B   DQ   0.698   0.655nH   0.668pF
Y5   VSS   GND   NA   NA   NA
Y8   VSS   GND   NA   NA   NA
Y9   DQ14_B   DQ   0.691   0.653nH   0.672pF
Y10   DMI1_B   DQ   0.819   0.738nH   0.735pF
Y11   DQ9_B   DQ   0.688   0.642nH   0.676pF
Y12   VSS   GND   NA   NA   NA
AA2   DQ0_B   DQ   0.709   0.697nH   0.668pF
AA3   VDDQ   POWER   NA   NA   NA
AA4   DQ7_B   DQ   0.735   0.700nH   0.660pF
AA5   VDDQ   POWER   NA   NA   NA
AA8   VDDQ   POWER   NA   NA   NA
AA9   DQ15_B   DQ   0.709   0.666nH   0.683pF
AA10   VDDQ   POWER   NA   NA   NA
AA11   DQ8_B   DQ   0.716   0.695nH   0.675pF
AB3   VSS   GND   NA   NA   NA
AB4   VDD2   POWER   NA   NA   NA
AB5   VSS   GND   NA   NA   NA
AB8   VSS   GND   NA   NA   NA
AB9   VDD2   POWER   NA   NA   NA
AB10   VSS   GND   NA   NA   NA
AB11   ERR_B   ERR   2.340   2.010nH   3.990pF
|IN   dq_in   dummy
|EN   dq_en   dummy
[Diff pin]  inv_pin  vdiff   tdelay_typ   tdelay_min   tdelay_max
D3   E3   0.180V   NA   NA   NA
D10   E10   0.180V   NA   NA   NA
J8   J9   0.180V   NA   NA   NA
P8   P9   0.180V   NA   NA   NA
W3   V3   0.180V   NA   NA   NA
W10   V10   0.180V   NA   NA   NA
[Model Selector] DQ
DQ_SOC40_PD40_VOH3  SocODT=RZQ/6, Pull-down=RZQ/6,PU-Cal at vddq/3
DQ_SOC48_PD40_VOH3  SocODT=RZQ/5, Pull-down=RZQ/6,PU-Cal at vddq/3
DQ_SOC60_PD40_VOH3  SocODT=RZQ/4, Pull-down=RZQ/6,PU-Cal at vddq/3
DQ_SOC80_PD40_VOH3  SocODT=RZQ/3, Pull-down=RZQ/6,PU-Cal at vddq/3
DQ_SOC120_PD40_VOH3  SocODT=RZQ/2, Pull-down=RZQ/6,PU-Cal at vddq/3
DQ_SOC240_PD40_VOH3  SocODT=RZQ/1, Pull-down=RZQ/6,PU-Cal at vddq/3
DQ_SOC40_PD60_VOH3  SocODT=RZQ/6, Pull-down=RZQ/6,PU-Cal at vddq/3
DQ_SOC48_PD60_VOH3  SocODT=RZQ/5, Pull-down=RZQ/6,PU-Cal at vddq/3
DQ_SOC60_PD60_VOH3  SocODT=RZQ/4, Pull-down=RZQ/6,PU-Cal at vddq/3
DQ_SOC80_PD60_VOH3  SocODT=RZQ/3, Pull-down=RZQ/6,PU-Cal at vddq/3
DQ_SOC120_PD60_VOH3  SocODT=RZQ/2, Pull-down=RZQ/6,PU-Cal at vddq/3
DQ_SOC240_PD60_VOH3  SocODT=RZQ/1, Pull-down=RZQ/6,PU-Cal at vddq/3
DQ_SOC40_PD48_VOH3  SocODT=RZQ/6, Pull-down=RZQ/6,PU-Cal at vddq/3
DQ_SOC48_PD48_VOH3  SocODT=RZQ/5, Pull-down=RZQ/6,PU-Cal at vddq/3
DQ_SOC60_PD48_VOH3  SocODT=RZQ/4, Pull-down=RZQ/6,PU-Cal at vddq/3
DQ_SOC80_PD48_VOH3  SocODT=RZQ/3, Pull-down=RZQ/6,PU-Cal at vddq/3
DQ_SOC120_PD48_VOH3  SocODT=RZQ/2, Pull-down=RZQ/6,PU-Cal at vddq/3
DQ_SOC240_PD48_VOH3  SocODT=RZQ/1, Pull-down=RZQ/6,PU-Cal at vddq/3
DQ_SOC40_PD80_VOH3  SocODT=RZQ/6, Pull-down=RZQ/6,PU-Cal at vddq/3
DQ_SOC48_PD80_VOH3  SocODT=RZQ/5, Pull-down=RZQ/6,PU-Cal at vddq/3
DQ_SOC60_PD80_VOH3  SocODT=RZQ/4, Pull-down=RZQ/6,PU-Cal at vddq/3
DQ_SOC80_PD80_VOH3  SocODT=RZQ/3, Pull-down=RZQ/6,PU-Cal at vddq/3
DQ_SOC120_PD80_VOH3  SocODT=RZQ/2, Pull-down=RZQ/6,PU-Cal at vddq/3
DQ_SOC240_PD80_VOH3  SocODT=RZQ/1, Pull-down=RZQ/6,PU-Cal at vddq/3
DQ_SOC40_PD120_VOH3  SocODT=RZQ/6, Pull-down=RZQ/6,PU-Cal at vddq/3
DQ_SOC48_PD120_VOH3  SocODT=RZQ/5, Pull-down=RZQ/6,PU-Cal at vddq/3
DQ_SOC60_PD120_VOH3  SocODT=RZQ/4, Pull-down=RZQ/6,PU-Cal at vddq/3
DQ_SOC80_PD120_VOH3  SocODT=RZQ/3, Pull-down=RZQ/6,PU-Cal at vddq/3
DQ_SOC120_PD120_VOH3  SocODT=RZQ/2, Pull-down=RZQ/6,PU-Cal at vddq/3
DQ_SOC240_PD120_VOH3  SocODT=RZQ/1, Pull-down=RZQ/6,PU-Cal at vddq/3
DQ_SOC40_PD240_VOH3  SocODT=RZQ/6, Pull-down=RZQ/6,PU-Cal at vddq/3
DQ_SOC48_PD240_VOH3  SocODT=RZQ/5, Pull-down=RZQ/6,PU-Cal at vddq/3
DQ_SOC60_PD240_VOH3  SocODT=RZQ/4, Pull-down=RZQ/6,PU-Cal at vddq/3
DQ_SOC80_PD240_VOH3  SocODT=RZQ/3, Pull-down=RZQ/6,PU-Cal at vddq/3
DQ_SOC120_PD240_VOH3  SocODT=RZQ/2, Pull-down=RZQ/6,PU-Cal at vddq/3
DQ_SOC240_PD240_VOH3  SocODT=RZQ/1, Pull-down=RZQ/6,PU-Cal at vddq/3
DQ_SOC80_PD40_VOH25  SocODT=RZQ/3, Pull-down=RZQ/6,PU-Cal at vddq/2.5
DQ_SOC80_PD48_VOH25  SocODT=RZQ/3, Pull-down=RZQ/5,PU-Cal at vddq/2.5
DQ_SOC80_PD60_VOH25  SocODT=RZQ/3, Pull-down=RZQ/4,PU-Cal at vddq/2.5
DQ_SOC80_PD80_VOH25  SocODT=RZQ/3, Pull-down=RZQ/3,PU-Cal at vddq/2.5
DQ_SOC80_PD120_VOH25  SocODT=RZQ/3, Pull-down=RZQ/2,PU-Cal at vddq/2.5
DQ_SOC80_PD240_VOH25  SocODT=RZQ/3, Pull-down=RZQ/1,PU-Cal at vddq/2.5
DQ_SOC120_PD40_VOH25  SocODT=RZQ/2, Pull-down=RZQ/6,PU-Cal at vddq/2.5
DQ_SOC120_PD48_VOH25  SocODT=RZQ/2, Pull-down=RZQ/5,PU-Cal at vddq/2.5
DQ_SOC120_PD60_VOH25  SocODT=RZQ/2, Pull-down=RZQ/4,PU-Cal at vddq/2.5
DQ_SOC120_PD80_VOH25  SocODT=RZQ/2, Pull-down=RZQ/3,PU-Cal at vddq/2.5
DQ_SOC120_PD120_VOH25  SocODT=RZQ/2, Pull-down=RZQ/2,PU-Cal at vddq/2.5
DQ_SOC120_PD240_VOH25  SocODT=RZQ/2, Pull-down=RZQ/1,PU-Cal at vddq/2.5
DQ_SOC240_PD40_VOH25  SocODT=RZQ/1, Pull-down=RZQ/6,PU-Cal at vddq/2.5
DQ_SOC240_PD48_VOH25  SocODT=RZQ/1, Pull-down=RZQ/5,PU-Cal at vddq/2.5
DQ_SOC240_PD60_VOH25  SocODT=RZQ/1, Pull-down=RZQ/4,PU-Cal at vddq/2.5
DQ_SOC240_PD80_VOH25  SocODT=RZQ/1, Pull-down=RZQ/3,PU-Cal at vddq/2.5
DQ_SOC240_PD120_VOH25  SocODT=RZQ/1, Pull-down=RZQ/2,PU-Cal at vddq/2.5
DQ_SOC240_PD240_VOH25  SocODT=RZQ/1, Pull-down=RZQ/1,PU-Cal at vddq/2.5
DQ_RCV_ODTOFF  DQ Input with no ODT
DQ_RCV_ODT40_VOH25  DQ Input with ODT 40 Ohm (RZQ/6),PU-Cal at vddq/2.5
DQ_RCV_ODT48_VOH25  DQ Input with ODT 48 Ohm (RZQ/5),PU-Cal at vddq/2.5
DQ_RCV_ODT60_VOH25  DQ Input with ODT 60 Ohm (RZQ/4),PU-Cal at vddq/2.5
DQ_RCV_ODT80_VOH25  DQ Input with ODT 80 Ohm (RZQ/3),PU-Cal at vddq/2.5
DQ_RCV_ODT120_VOH25  DQ Input with ODT 120 Ohm (RZQ/2),PU-Cal at vddq/2.5
DQ_RCV_ODT240_VOH25  DQ Input with ODT 240 Ohm (RZQ/1),PU-Cal at vddq/2.5
DQ_RCV_ODT40_VOH3  DQ Input with ODT 40 Ohm (RZQ/6),PU-Cal at vddq/3
DQ_RCV_ODT48_VOH3  DQ Input with ODT 48 Ohm (RZQ/5),PU-Cal at vddq/3
DQ_RCV_ODT60_VOH3  DQ Input with ODT 60 Ohm (RZQ/4),PU-Cal at vddq/3
DQ_RCV_ODT80_VOH3  DQ Input with ODT 80 Ohm (RZQ/3),PU-Cal at vddq/3
DQ_RCV_ODT120_VOH3  DQ Input with ODT 120 Ohm (RZQ/2),PU-Cal at vddq/3
DQ_RCV_ODT240_VOH3  DQ Input with ODT 240 Ohm (RZQ/1),PU-Cal at vddq/3
[Model Selector] CLKCA
CLKCA_RCV_ODTOFF  CA Input with ODT OFF
CLKCA_RCV_ODT40_VOH3  CA Input with ODT 40 Ohm (RZQ/6),PU-Cal at vddq/3
CLKCA_RCV_ODT48_VOH3  CA Input with ODT 48 Ohm (RZQ/5),PU-Cal at vddq/3
CLKCA_RCV_ODT60_VOH3  CA Input with ODT 60 Ohm (RZQ/4),PU-Cal at vddq/3
CLKCA_RCV_ODT80_VOH3  CA Input with ODT 80 Ohm (RZQ/3),PU-Cal at vddq/3
CLKCA_RCV_ODT120_VOH3  CA Input with ODT 120 Ohm (RZQ/2),PU-Cal at vddq/3
CLKCA_RCV_ODT240_VOH3  CA Input with ODT 240 Ohm (RZQ/1),PU-Cal at vddq/3
CLKCA_RCV_ODT40_VOH25  CA Input with ODT 40 Ohm (RZQ/6),PU-Cal at vddq/2.5
CLKCA_RCV_ODT48_VOH25  CA Input with ODT 48 Ohm (RZQ/5),PU-Cal at vddq/2.5
CLKCA_RCV_ODT60_VOH25  CA Input with ODT 60 Ohm (RZQ/4),PU-Cal at vddq/2.5
CLKCA_RCV_ODT80_VOH25  CA Input with ODT 80 Ohm (RZQ/3),PU-Cal at vddq/2.5
CLKCA_RCV_ODT120_VOH25  CA Input with ODT 120 Ohm (RZQ/2),PU-Cal at vddq/2.5
CLKCA_RCV_ODT240_VOH25  CA Input with ODT 240 Ohm (RZQ/1),PU-Cal at vddq/2.5
| Models and submodels in the file (94): DQ_SOC40_PD40_VOH3 (I/O), DQ_SOC40_PD48_VOH3 (I/O), DQ_SOC40_PD60_VOH3 (I/O), DQ_SOC40_PD80_VOH3 (I/O), DQ_SOC40_PD120_VOH3 (I/O), DQ_SOC40_PD240_VOH3 (I/O), DQ_SOC48_PD40_VOH3 (I/O), DQ_SOC48_PD48_VOH3 (I/O), DQ_SOC48_PD60_VOH3 (I/O), DQ_SOC48_PD80_VOH3 (I/O), DQ_SOC48_PD120_VOH3 (I/O), DQ_SOC48_PD240_VOH3 (I/O), DQ_SOC60_PD40_VOH3 (I/O), DQ_SOC60_PD48_VOH3 (I/O), DQ_SOC60_PD60_VOH3 (I/O), DQ_SOC60_PD80_VOH3 (I/O), DQ_SOC60_PD120_VOH3 (I/O), DQ_SOC60_PD240_VOH3 (I/O), DQ_SOC80_PD40_VOH3 (I/O), DQ_SOC80_PD48_VOH3 (I/O), DQ_SOC80_PD60_VOH3 (I/O), DQ_SOC80_PD80_VOH3 (I/O), DQ_SOC80_PD120_VOH3 (I/O), DQ_SOC80_PD240_VOH3 (I/O), DQ_SOC120_PD40_VOH3 (I/O), DQ_SOC120_PD48_VOH3 (I/O), DQ_SOC120_PD60_VOH3 (I/O), DQ_SOC120_PD80_VOH3 (I/O), DQ_SOC120_PD120_VOH3 (I/O), DQ_SOC120_PD240_VOH3 (I/O), DQ_SOC240_PD40_VOH3 (I/O), DQ_SOC240_PD48_VOH3 (I/O), DQ_SOC240_PD60_VOH3 (I/O), DQ_SOC240_PD80_VOH3 (I/O), DQ_SOC240_PD120_VOH3 (I/O), DQ_SOC240_PD240_VOH3 (I/O), DQ_SOC80_PD40_VOH25 (I/O), DQ_SOC80_PD48_VOH25 (I/O), DQ_SOC80_PD60_VOH25 (I/O), DQ_SOC80_PD80_VOH25 (I/O), DQ_SOC80_PD120_VOH25 (I/O), DQ_SOC80_PD240_VOH25 (I/O), DQ_SOC120_PD40_VOH25 (I/O), DQ_SOC120_PD48_VOH25 (I/O), DQ_SOC120_PD60_VOH25 (I/O), DQ_SOC120_PD80_VOH25 (I/O), DQ_SOC120_PD120_VOH25 (I/O), DQ_SOC120_PD240_VOH25 (I/O), DQ_SOC240_PD40_VOH25 (I/O), DQ_SOC240_PD48_VOH25 (I/O), DQ_SOC240_PD60_VOH25 (I/O), DQ_SOC240_PD80_VOH25 (I/O), DQ_SOC240_PD120_VOH25 (I/O), DQ_SOC240_PD240_VOH25 (I/O), DQ_RCV_ODTOFF (Input), DQ_RCV_ODT40_VOH3 (Input), DQ_RCV_ODT48_VOH3 (Input), DQ_RCV_ODT60_VOH3 (Input), DQ_RCV_ODT80_VOH3 (Input), DQ_RCV_ODT120_VOH3 (Input), DQ_RCV_ODT240_VOH3 (Input), DQ_RCV_ODT40_VOH25 (Input), DQ_RCV_ODT48_VOH25 (Input), DQ_RCV_ODT60_VOH25 (Input), DQ_RCV_ODT80_VOH25 (Input), DQ_RCV_ODT120_VOH25 (Input), DQ_RCV_ODT240_VOH25 (Input), CLKCA_RCV_ODTOFF (Input), CLKCA_RCV_ODT40_VOH3 (Input), CLKCA_RCV_ODT48_VOH3 (Input), CLKCA_RCV_ODT60_VOH3 (Input), CLKCA_RCV_ODT80_VOH3 (Input), CLKCA_RCV_ODT120_VOH3 (Input), CLKCA_RCV_ODT240_VOH3 (Input), CLKCA_RCV_ODT40_VOH25 (Input), CLKCA_RCV_ODT48_VOH25 (Input), CLKCA_RCV_ODT60_VOH25 (Input), CLKCA_RCV_ODT80_VOH25 (Input), CLKCA_RCV_ODT120_VOH25 (Input), CLKCA_RCV_ODT240_VOH25 (Input)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
